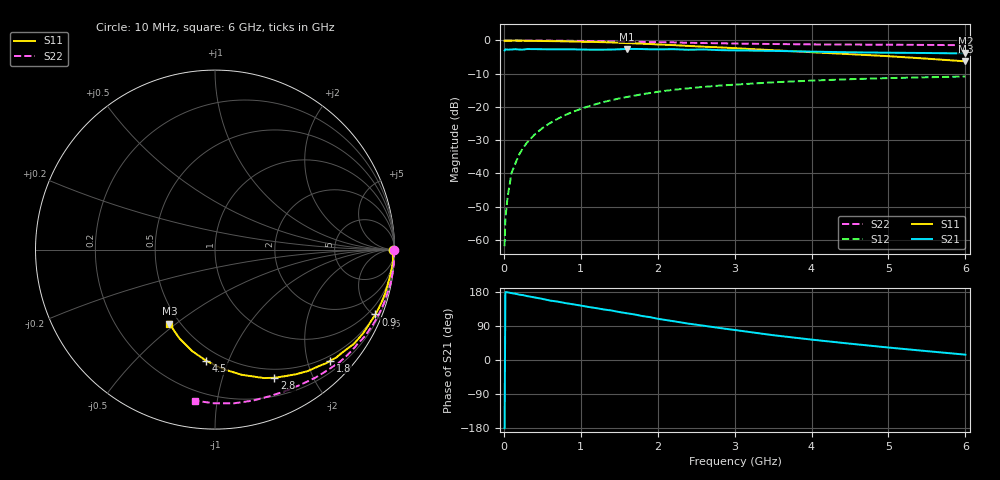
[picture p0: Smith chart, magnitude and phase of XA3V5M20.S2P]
! SIEMENS Discrete & RF Semiconductors
! BFY180
! Si NPN RF Bipolar Junction Transistor in MICRO-X
! VCE = 3.5 V  IC = 0.2 mA
! Common Emitter S-Parameters:  May  1997
# GHz  S  MA  R  50
!  f  S11  S21  S12  S22
! GHz  MAG  ANG  MAG  ANG  MAG  ANG  MAG  ANG
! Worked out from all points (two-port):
!   36 points, 10 MHz to 6 GHz, reference 50 ohm
!   highest |S21| = -2.56 dB at 1.6 GHz (marker M1); lowest = -3.9 dB at 6 GHz (marker M2)
!   |S21| within 3 dB of the highest: start of sweep to end of sweep
!   lowest |S11| = -6.3 dB at 6 GHz (marker M3), VSWR 2.88, Z = 21.9 - j23.6 ohm
!   |S11| at or under -10 dB: nowhere
!   |S22| runs from -1.4 to 0.0 dB; largest |S21 - S12| = 0.74
!   S11 on the Smith chart (normalised r, x): 10 MHz: open; 900 MHz: 0.50, -5.10; 1.8 GHz: 0.40, -2.43; 2.8 GHz: 0.40, -1.49; 4.5 GHz: 0.41, -0.84; 6 GHz: 0.44, -0.47
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0.01  0.9901 -0.1  0.707 -180.0  0.0008 82.6  0.9993 -0.2
0.02  0.9886 -0.2  0.735 179.1  0.0021 93.3  0.9999 -0.5
0.05  0.9907 -1.0  0.728 178.5  0.0045 89.1  0.9991 -1.0
0.1  0.9921 -2.5  0.73 176.5  0.0101 87.4  0.9983 -2.0
0.2  0.9918 -4.8  0.729 172.5  0.0193 86.7  0.9986 -4.0
0.3  0.9887 -7.2  0.742 168.7  0.0289 83.9  0.9975 -5.9
0.4  0.9842 -9.8  0.741 165.1  0.0384 81.7  0.9977 -7.9
0.5  0.9804 -12.5  0.737 161.3  0.0478 79.1  0.9968 -9.9
0.7  0.9738 -17.3  0.736 154.1  0.0662 74.9  0.991 -13.9
0.9  0.964 -22.0  0.735 147.0  0.0844 70.3  0.9872 -17.9
1.1  0.9519 -26.8  0.728 140.0  0.1018 66.4  0.9806 -21.8
1.3  0.9407 -31.9  0.728 133.3  0.1188 62.0  0.9738 -25.6
1.6  0.9117 -39.1  0.745 123.2  0.1409 56.1  0.96 -31.4
1.8  0.8925 -43.9  0.742 116.0  0.1552 52.3  0.9504 -34.9
2.2  0.8518 -52.6  0.739 102.5  0.1805 44.5  0.9354 -42.1
2.6  0.8047 -61.3  0.733 90.4  0.2001 37.7  0.9147 -48.5
2.8  0.787 -65.2  0.715 84.6  0.209 34.6  0.9072 -51.6
3.5  0.713 -78.0  0.697 65.5  0.2343 24.4  0.8837 -61.8
4  0.6658 -86.4  0.679 53.8  0.2485 17.7  0.8726 -68.9
4.5  0.6215 -94.5  0.663 43.1  0.2612 11.6  0.8674 -75.9
5.5  0.5321 -112.0  0.647 23.4  0.2793 -0.1  0.8564 -90.3
6  0.4844 -121.7  0.637 14.1  0.2861 -6.2  0.849 -97.5
